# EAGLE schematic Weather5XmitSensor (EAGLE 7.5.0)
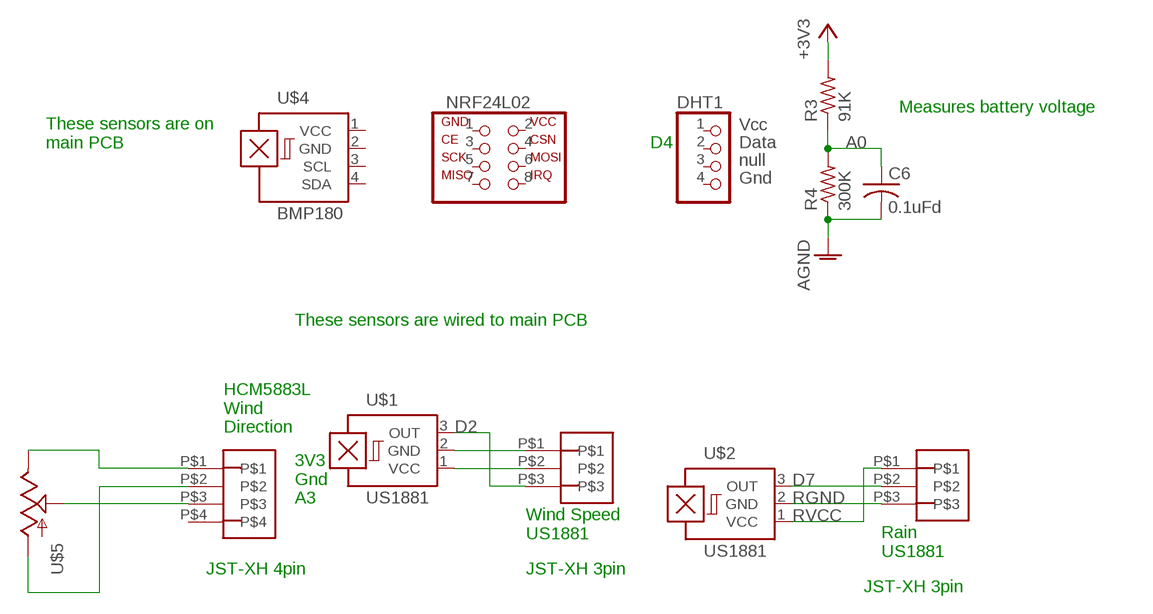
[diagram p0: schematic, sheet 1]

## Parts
C6  0.1uFd  C-US025-025X050  [C025-025X050]
DHT1  DHT22  [1X04]
HCM5883L  4_PIN_JST-XH  [4_PIN_JST-XH]
NRF24L02  NRF24L01+  [NRF24L01+]
R3  91K  R-US_0204/7  [0204/7]
R4  300K  R-US_0207/2V  [0207/2V]
RAIN  3_PIN_JST-XH  [3_PIN_JST-XH]
U$1  US1881  [US1881]
U$2  US1881  [US1881]
U$4  BMP180  [BMP180]
U$5  POT100K_3362U  [3362U]
WSPEED  3_PIN_JST-XH  [3_PIN_JST-XH]

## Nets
+3V3: R3.2
A0: C6.1 R3.1 R4.2
AGND [power]: C6.2 R4.1
D2: U$1.3(OUT) WSPEED.P$3
D7: RAIN.P$2 U$2.3(OUT)
N$2: U$1.1(VCC) WSPEED.P$2
N$3: HCM5883L.P$1 U$5.P$1(E)
N$4: HCM5883L.P$2 U$5.P$3(A)
N$5 [power]: U$1.2(GND) WSPEED.P$1
N$7: HCM5883L.P$3 U$5.P$2(S)
RGND: RAIN.P$3 U$2.2(GND)
RVCC: RAIN.P$1 U$2.1(VCC)
Unconnected: DHT1.1(VCC) DHT1.2(DATA) DHT1.3(NULL) DHT1.4(GND) HCM5883L.P$4 NRF24L02.1 NRF24L02.2 NRF24L02.3 NRF24L02.4 NRF24L02.5 NRF24L02.6 NRF24L02.7 NRF24L02.8 U$4.3(SCL) U$4.4(SDA)

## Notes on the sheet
- Measures battery voltage
- These sensors are on
  main PCB
- D4
- These sensors are wired to main PCB
- HCM5883L
  Wind
  Direction
- 3V3
  Gnd
  A3
- Wind Speed
  US1881
- Rain
  US1881
- JST-XH 4pin | JST-XH 3pin
- JST-XH 3pin

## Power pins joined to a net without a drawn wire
GND: U$4.2(GND)
VCC: U$4.1(VCC)

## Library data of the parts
C6 = MTS:C-US: CAPACITOR, American symbol
DHT1 = MTS_Custom:DHT22
HCM5883L = JST-XH_HEADERS:4_PIN_JST-XH
NRF24L02 = MTS_Custom:NRF24L01+
R3 R4 = MTS:R-US_: RESISTOR, American symbol
RAIN WSPEED = JST-XH_HEADERS:3_PIN_JST-XH
U$1 U$2 = MTS_Custom:US1881: Hall Effect bipolar latching sensor
U$4 = MTS_Custom:BMP180: This is a Bosch BMP180 pressure sensor
U$5 = SparkFun:POT

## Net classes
0 default: width 0.4 mm, clearance 0.3 mm
1 power: width 0.6 mm, clearance 0.3 mm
